(* Logix 5000 Program export KEP; software revision 30.00; part 7 of 15 *)

ADD_ON_INSTRUCTION B256_DEC   (* revision 1.0 20170916, vendor Kenneth A. Fischer *)
// c1 = --c1
// Revision note:
// Rev1.0: 20170916 - Initial Release
VAR_IN_OUT
   Inp_C : DINT[22]; {required}
END_VAR
VAR
   i : DINT;
END_VAR

ROUTINE Logic   (* ladder *)
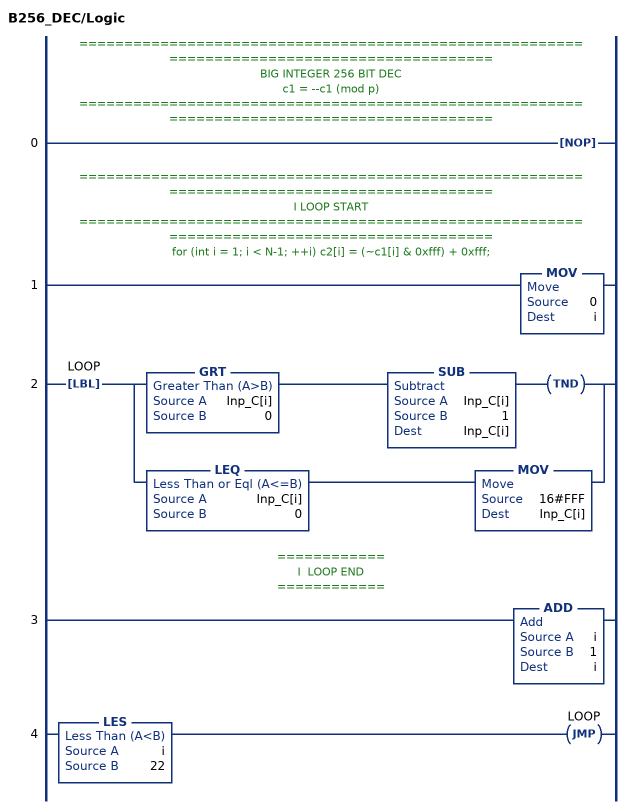
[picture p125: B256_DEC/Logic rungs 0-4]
   // ============================================================================================
   // BIG INTEGER 256 BIT DEC
   // c1 = --c1 (mod p)
   // ============================================================================================
   0: NOP();
   // ============================================================================================
   // I LOOP START
   // ============================================================================================
   // for (int i = 1; i < N-1; ++i) c2[i] = (~c1[i] & 0xfff) + 0xfff;
   1: MOV(0,i);
   2: LBL(LOOP)[GRT(Inp_C[i],0) SUB(Inp_C[i],1,Inp_C[i]) TND() ,LEQ(Inp_C[i],0) MOV(16#FFF,Inp_C[i]) ];
   // ============
   // I  LOOP END
   // ============
   3: ADD(i,1,i);
   4: LES(i,22)JMP(LOOP);
END_ROUTINE
END_ADD_ON_INSTRUCTION

ADD_ON_INSTRUCTION B256_MODPOW   (* revision 1.0 20170916, vendor Kenneth A. Fischer *)
// c2 = c1^e mod (2^255-19)
// Revision note:
// Rev1.0: 20170916 - Initial Release
VAR_IN_OUT
   Temp_C1 : DINT[22]; {required}
   Temp_C2 : DINT[22]; {required}
   Temp_D : DINT[43]; {required}
   Inp_C1 : DINT[22]; {required}   // V
   Inp_E : DINT[32]; {required}
   Out_C2 : DINT[22]; {required}   // U
END_VAR
VAR_OUTPUT
   i : INT; {access Read Only}
END_VAR
VAR_INPUT
   SEQCTRL_RESET : BOOL;   // Resets Point Multiplication if Toggled True
END_VAR
VAR_OUTPUT
   SEQCTRL_DN : BOOL; {access Read Only}   // Complete
   SEQCTRL_STEP : INT; {access Read Only}
END_VAR
VAR
   SEQCTRL_CMD : INT;
   SEQCTRL_DONE : INT;
   SEQCTRL_CMD_TABLE : INT[35];
   SEQCTRL_NEXT_STEP : INT;
   TEMP : INT;
   j : INT;
   b : DINT;
   B256_MUL : B256_MUL;
   B256_SQU : B256_SQU;
END_VAR

ROUTINE Logic   (* ladder *)
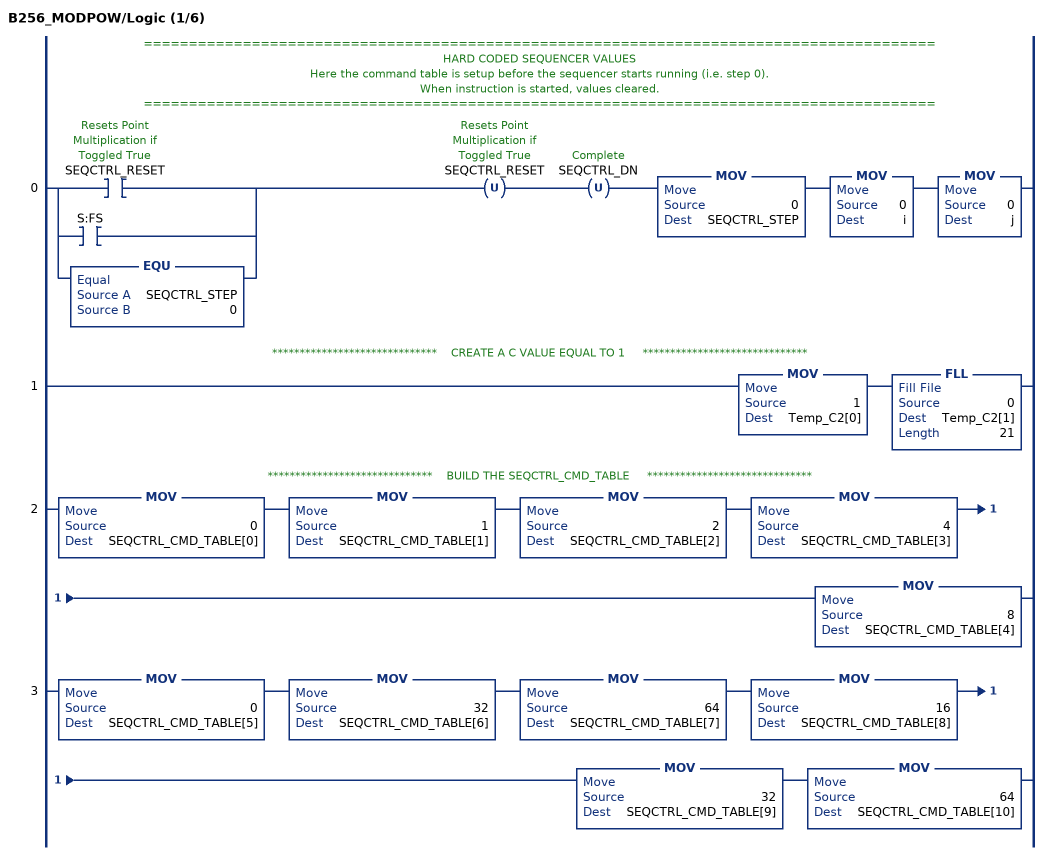
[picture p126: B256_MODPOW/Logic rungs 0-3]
   // ========================================================================================
   // HARD CODED SEQUENCER VALUES
   // Here the command table is setup before the sequencer starts running (i.e. step 0).
   // When instruction is started, values cleared.
   // ========================================================================================
   0: [[XIC(SEQCTRL_RESET) ,XIC(S:FS) ] ,EQU(SEQCTRL_STEP,0) ]OTU(SEQCTRL_RESET)OTU(SEQCTRL_DN)MOV(0,SEQCTRL_STEP)MOV(0,i)MOV(0,j);
   // ******************************    CREATE A C VALUE EQUAL TO 1     ******************************
   1: MOV(1,Temp_C2[0])FLL(0,Temp_C2[1],21);
   // ******************************    BUILD THE SEQCTRL_CMD_TABLE     ******************************
   2: MOV(0,SEQCTRL_CMD_TABLE[0])MOV(1,SEQCTRL_CMD_TABLE[1])MOV(2,SEQCTRL_CMD_TABLE[2])MOV(4,SEQCTRL_CMD_TABLE[3])MOV(8,SEQCTRL_CMD_TABLE[4]);
   3: MOV(0,SEQCTRL_CMD_TABLE[5])MOV(32,SEQCTRL_CMD_TABLE[6])MOV(64,SEQCTRL_CMD_TABLE[7])MOV(16,SEQCTRL_CMD_TABLE[8])MOV(32,SEQCTRL_CMD_TABLE[9])MOV(64,SEQCTRL_CMD_TABLE[10]);
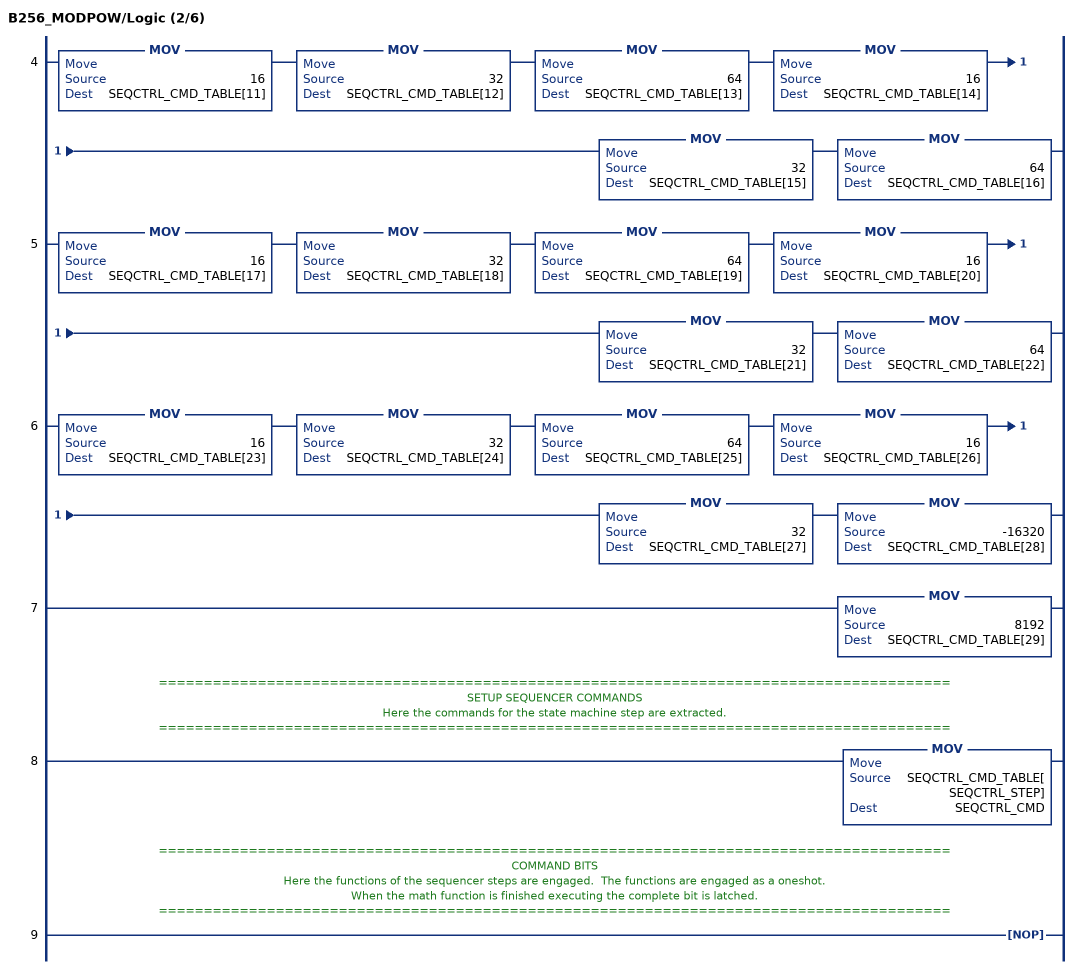
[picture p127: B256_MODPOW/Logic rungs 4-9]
   4: MOV(16,SEQCTRL_CMD_TABLE[11])MOV(32,SEQCTRL_CMD_TABLE[12])MOV(64,SEQCTRL_CMD_TABLE[13])MOV(16,SEQCTRL_CMD_TABLE[14])MOV(32,SEQCTRL_CMD_TABLE[15])MOV(64,SEQCTRL_CMD_TABLE[16]);
   5: MOV(16,SEQCTRL_CMD_TABLE[17])MOV(32,SEQCTRL_CMD_TABLE[18])MOV(64,SEQCTRL_CMD_TABLE[19])MOV(16,SEQCTRL_CMD_TABLE[20])MOV(32,SEQCTRL_CMD_TABLE[21])MOV(64,SEQCTRL_CMD_TABLE[22]);
   6: MOV(16,SEQCTRL_CMD_TABLE[23])MOV(32,SEQCTRL_CMD_TABLE[24])MOV(64,SEQCTRL_CMD_TABLE[25])MOV(16,SEQCTRL_CMD_TABLE[26])MOV(32,SEQCTRL_CMD_TABLE[27])MOV(-16320,SEQCTRL_CMD_TABLE[28]);
   7: MOV(8192,SEQCTRL_CMD_TABLE[29]);
   // ========================================================================================
   // SETUP SEQUENCER COMMANDS
   // Here the commands for the state machine step are extracted.
   // ========================================================================================
   8: MOV(SEQCTRL_CMD_TABLE[SEQCTRL_STEP],SEQCTRL_CMD);
   // ========================================================================================
   // COMMAND BITS
   // Here the functions of the sequencer steps are engaged.  The functions are engaged as a oneshot.
   // When the math function is finished executing the complete bit is latched.
   // ========================================================================================
   9: NOP();
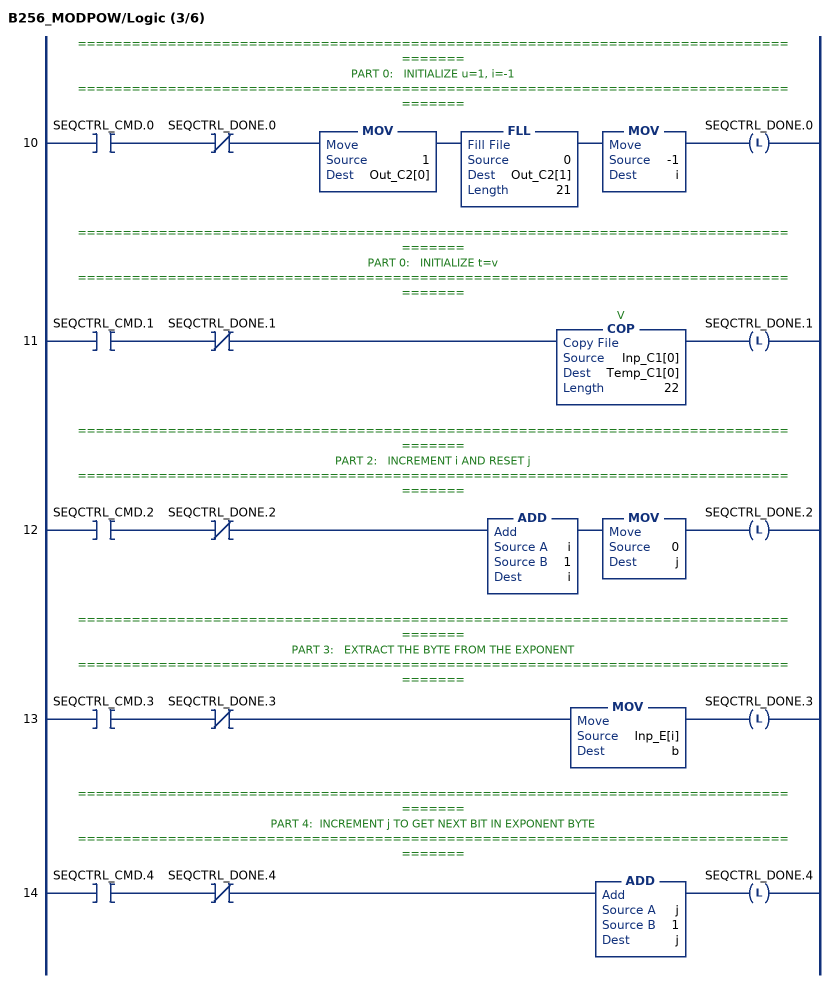
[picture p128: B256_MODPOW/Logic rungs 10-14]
   // ======================================================================================
   // PART 0:   INITIALIZE u=1, i=-1
   // ======================================================================================
   10: XIC(SEQCTRL_CMD.0)XIO(SEQCTRL_DONE.0)MOV(1,Out_C2[0])FLL(0,Out_C2[1],21)MOV(-1,i)OTL(SEQCTRL_DONE.0);
   // ======================================================================================
   // PART 0:   INITIALIZE t=v
   // ======================================================================================
   11: XIC(SEQCTRL_CMD.1)XIO(SEQCTRL_DONE.1)COP(Inp_C1[0],Temp_C1[0],22)OTL(SEQCTRL_DONE.1);
   // ======================================================================================
   // PART 2:   INCREMENT i AND RESET j
   // ======================================================================================
   12: XIC(SEQCTRL_CMD.2)XIO(SEQCTRL_DONE.2)ADD(i,1,i)MOV(0,j)OTL(SEQCTRL_DONE.2);
   // ======================================================================================
   // PART 3:   EXTRACT THE BYTE FROM THE EXPONENT
   // ======================================================================================
   13: XIC(SEQCTRL_CMD.3)XIO(SEQCTRL_DONE.3)MOV(Inp_E[i],b)OTL(SEQCTRL_DONE.3);
   // ======================================================================================
   // PART 4:  INCREMENT j TO GET NEXT BIT IN EXPONENT BYTE
   // ======================================================================================
   14: XIC(SEQCTRL_CMD.4)XIO(SEQCTRL_DONE.4)ADD(j,1,j)OTL(SEQCTRL_DONE.4);
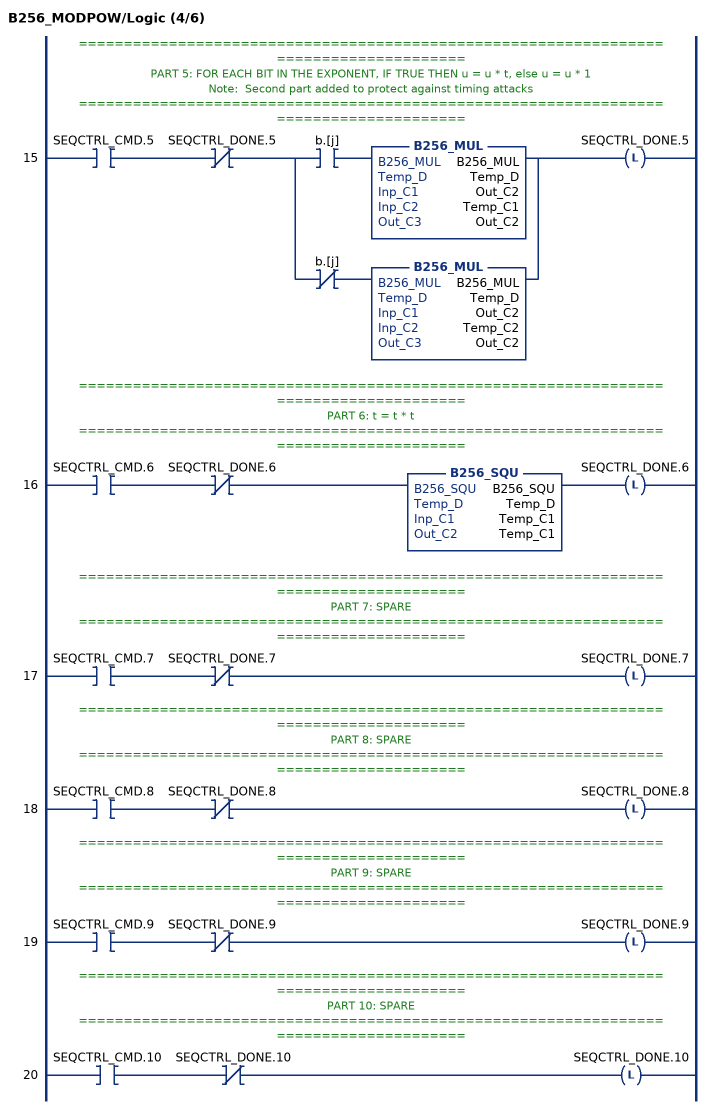
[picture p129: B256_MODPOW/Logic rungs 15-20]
   // ======================================================================================
   // PART 5: FOR EACH BIT IN THE EXPONENT, IF TRUE THEN u = u * t, else u = u * 1
   // Note:  Second part added to protect against timing attacks
   // ======================================================================================
   15: XIC(SEQCTRL_CMD.5)XIO(SEQCTRL_DONE.5)[XIC(b.[j]) B256_MUL(B256_MUL,Temp_D,Out_C2,Temp_C1,Out_C2) ,XIO(b.[j]) B256_MUL(B256_MUL,Temp_D,Out_C2,Temp_C2,Out_C2) ]OTL(SEQCTRL_DONE.5);
   // ======================================================================================
   // PART 6: t = t * t
   // ======================================================================================
   16: XIC(SEQCTRL_CMD.6)XIO(SEQCTRL_DONE.6)B256_SQU(B256_SQU,Temp_D,Temp_C1,Temp_C1)OTL(SEQCTRL_DONE.6);
   // ======================================================================================
   // PART 7: SPARE
   // ======================================================================================
   17: XIC(SEQCTRL_CMD.7)XIO(SEQCTRL_DONE.7)OTL(SEQCTRL_DONE.7);
   // ======================================================================================
   // PART 8: SPARE
   // ======================================================================================
   18: XIC(SEQCTRL_CMD.8)XIO(SEQCTRL_DONE.8)OTL(SEQCTRL_DONE.8);
   // ======================================================================================
   // PART 9: SPARE
   // ======================================================================================
   19: XIC(SEQCTRL_CMD.9)XIO(SEQCTRL_DONE.9)OTL(SEQCTRL_DONE.9);
   // ======================================================================================
   // PART 10: SPARE
   // ======================================================================================
   20: XIC(SEQCTRL_CMD.10)XIO(SEQCTRL_DONE.10)OTL(SEQCTRL_DONE.10);
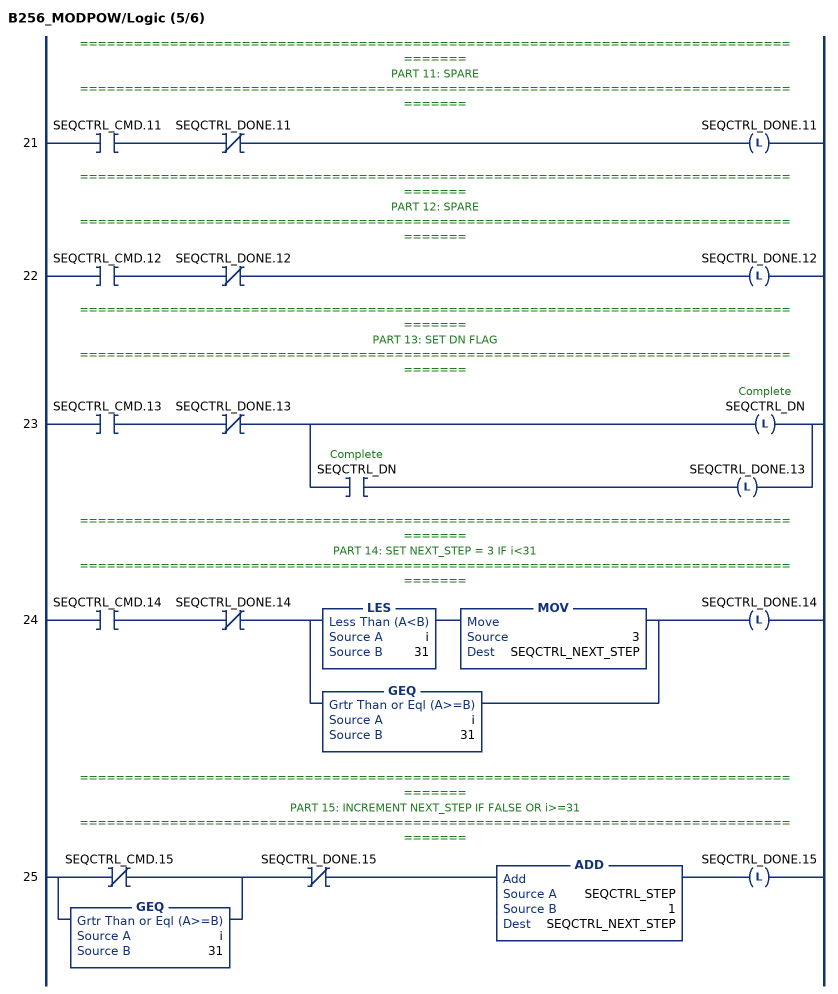
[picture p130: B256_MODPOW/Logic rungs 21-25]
   // ======================================================================================
   // PART 11: SPARE
   // ======================================================================================
   21: XIC(SEQCTRL_CMD.11)XIO(SEQCTRL_DONE.11)OTL(SEQCTRL_DONE.11);
   // ======================================================================================
   // PART 12: SPARE
   // ======================================================================================
   22: XIC(SEQCTRL_CMD.12)XIO(SEQCTRL_DONE.12)OTL(SEQCTRL_DONE.12);
   // ======================================================================================
   // PART 13: SET DN FLAG
   // ======================================================================================
   23: XIC(SEQCTRL_CMD.13)XIO(SEQCTRL_DONE.13)[OTL(SEQCTRL_DN) ,XIC(SEQCTRL_DN) OTL(SEQCTRL_DONE.13) ];
   // ======================================================================================
   // PART 14: SET NEXT_STEP = 3 IF i<31
   // ======================================================================================
   24: XIC(SEQCTRL_CMD.14)XIO(SEQCTRL_DONE.14)[LES(i,31) MOV(3,SEQCTRL_NEXT_STEP) ,GEQ(i,31) ]OTL(SEQCTRL_DONE.14);
   // ======================================================================================
   // PART 15: INCREMENT NEXT_STEP IF FALSE OR i>=31
   // ======================================================================================
   25: [XIO(SEQCTRL_CMD.15) ,GEQ(i,31) ]XIO(SEQCTRL_DONE.15)ADD(SEQCTRL_STEP,1,SEQCTRL_NEXT_STEP)OTL(SEQCTRL_DONE.15);
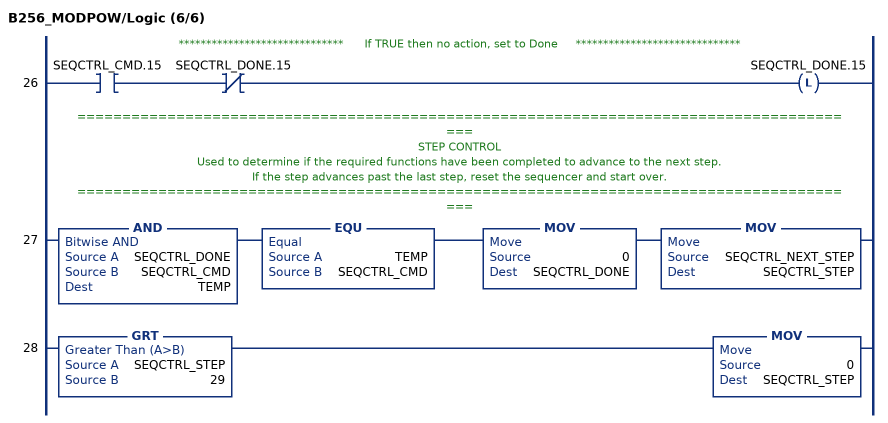
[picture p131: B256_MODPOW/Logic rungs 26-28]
   // ******************************      If TRUE then no action, set to Done     ******************************
   26: XIC(SEQCTRL_CMD.15)XIO(SEQCTRL_DONE.15)OTL(SEQCTRL_DONE.15);
   // ========================================================================================
   // STEP CONTROL
   // Used to determine if the required functions have been completed to advance to the next step.
   // If the step advances past the last step, reset the sequencer and start over.
   // ========================================================================================
   27: AND(SEQCTRL_DONE,SEQCTRL_CMD,TEMP)EQU(TEMP,SEQCTRL_CMD)MOV(0,SEQCTRL_DONE)MOV(SEQCTRL_NEXT_STEP,SEQCTRL_STEP);
   28: GRT(SEQCTRL_STEP,29)MOV(0,SEQCTRL_STEP);
END_ROUTINE
END_ADD_ON_INSTRUCTION

ADD_ON_INSTRUCTION B256_NEG   (* revision 1.0 20170916, vendor Kenneth A. Fischer *)
// c2 = -c1 (mod p)
// Revision note:
// Rev1.0: 20170916 - Initial Release
VAR_OUTPUT
   FAIL : BOOL; {access Read Only}   // Indicates negative overflow which should not happen
END_VAR
VAR_IN_OUT
   Inp_C1 : DINT[22]; {required}
   Out_C2 : DINT[22]; {required}
END_VAR
VAR
   s : DINT;
   b : DINT;
   i : DINT;
END_VAR

ROUTINE Logic   (* ladder *)
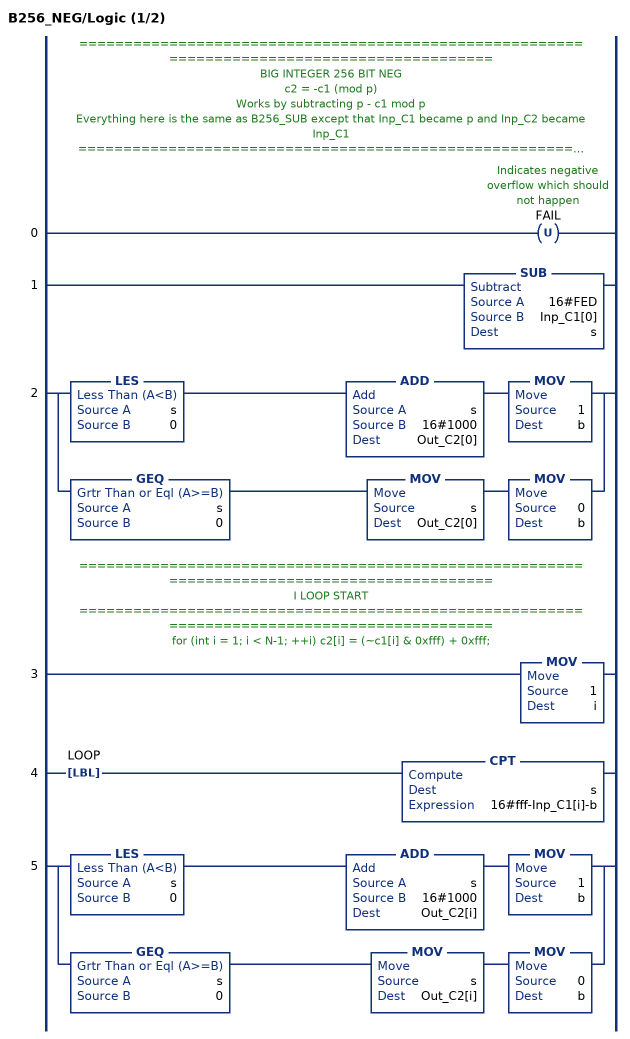
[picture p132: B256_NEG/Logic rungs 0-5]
   // ============================================================================================
   // BIG INTEGER 256 BIT NEG
   // c2 = -c1 (mod p)
   // Works by subtracting p - c1 mod p
   // Everything here is the same as B256_SUB except that Inp_C1 became p and Inp_C2 became Inp_C1
   // ============================================================================================
   0: OTU(FAIL);
   1: SUB(16#FED,Inp_C1[0],s);
   2: [LES(s,0) ADD(s,16#1000,Out_C2[0]) MOV(1,b) ,GEQ(s,0) MOV(s,Out_C2[0]) MOV(0,b) ];
   // ============================================================================================
   // I LOOP START
   // ============================================================================================
   // for (int i = 1; i < N-1; ++i) c2[i] = (~c1[i] & 0xfff) + 0xfff;
   3: MOV(1,i);
   4: LBL(LOOP)CPT(s,16#fff-Inp_C1[i]-b);
   5: [LES(s,0) ADD(s,16#1000,Out_C2[i]) MOV(1,b) ,GEQ(s,0) MOV(s,Out_C2[i]) MOV(0,b) ];
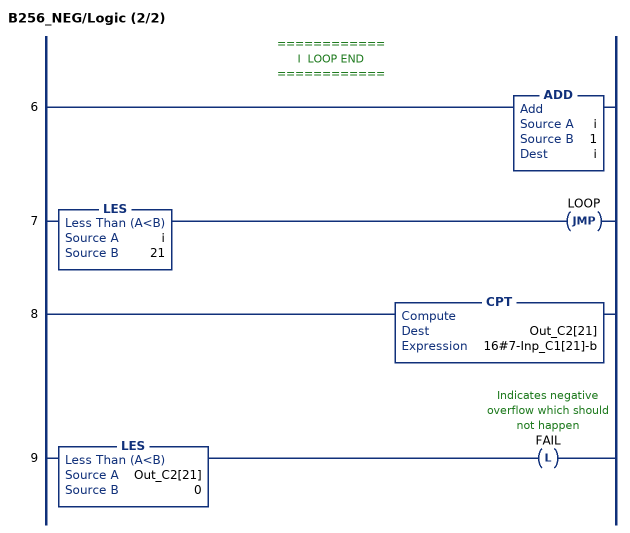
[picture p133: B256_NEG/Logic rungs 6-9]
   // ============
   // I  LOOP END
   // ============
   6: ADD(i,1,i);
   7: LES(i,21)JMP(LOOP);
   8: CPT(Out_C2[21],16#7-Inp_C1[21]-b);
   9: LES(Out_C2[21],0)OTL(FAIL);
END_ROUTINE
END_ADD_ON_INSTRUCTION

ADD_ON_INSTRUCTION POINT_DEC   (* revision 1.0 20170916, vendor Kenneth A. Fischer *)
// Point Decode:
// Decode a string value representing a point (x,y) into POINT data type in extended coordinates pieces
// Requires POINT UDT
// Revision note:
// Rev1.0: 20170916 - Initial Release
VAR_INPUT
   SEQCTRL_RESET : BOOL;   // Resets Point Multiplication if Toggled True
END_VAR
VAR_OUTPUT
   SEQCTRL_DN : BOOL; {access Read Only}   // Complete
   SEQCTRL_STEP : INT; {access Read Only}
   SEQCTRL_SUBSTEP : INT; {access Read Only}
   FAILED : BOOL; {access Read Only}
END_VAR
VAR_IN_OUT
   Temp_C1 : DINT[22]; {required}   // d
   Temp_C2 : DINT[22]; {required}   // m-1
   Temp_C3 : DINT[22]; {required}   // sqrtm1 = 2^((m-1)/4)
   Temp_C4 : DINT[22]; {required}   // u
   Temp_C5 : DINT[22]; {required}   // v
   Temp_C6 : DINT[22]; {required}   // v2
   Temp_C7 : DINT[22]; {required}   // v4
   Temp_C8 : DINT[22]; {required}   // t1
   Temp_C9 : DINT[22]; {required}   // t2
   Temp_C10 : DINT[22]; {required}   // t3
   Temp_C11 : DINT[22]; {required}
   Temp_C12 : DINT[22]; {required}
   Temp_D : DINT[43]; {required}
   Temp_E : DINT[32]; {required}   // m58 = (m-5)/8
   Inp_SLE : STRING; {required}   // Encoded Point as a String
   Out_P : POINT; {required}   // POINT in extended coordinates
END_VAR
VAR
   SEQCTRL_CMD : DINT;
   SEQCTRL_DONE : DINT;
   SEQCTRL_NEXT_STEP : INT;
   SEQCTRL_CMD_TABLE : DINT[40];
   TEMP : DINT;
   B256_StoC_LE : B256_StoC_LE;
   x_0 : BOOL;
   B256_SQU : B256_SQU;
   B256_SUB : B256_SUB;
   B256_MUL : B256_MUL;
   B256_ADD : B256_ADD;
   B256_MODPOW : B256_MODPOW;
   SEQCTRL_ONS : DINT;
   B256_COMPARE : B256_COMPARE;
   B256_NEG : B256_NEG;
   B256_COMPARE1 : B256_COMPARE;
   B256_COMPARE2 : B256_COMPARE;
   B256_ADJ : B256_ADJ;
   B256_DEC : B256_DEC;
END_VAR

ROUTINE Logic   (* ladder *)
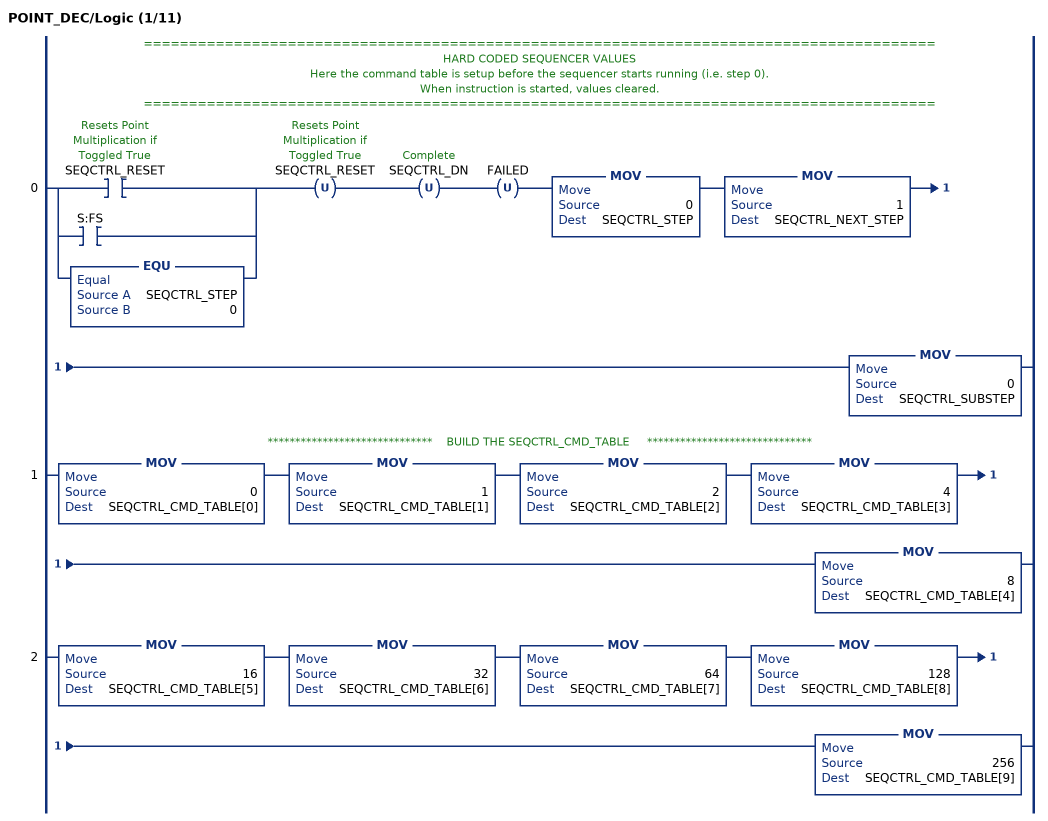
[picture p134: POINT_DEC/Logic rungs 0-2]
   // ========================================================================================
   // HARD CODED SEQUENCER VALUES
   // Here the command table is setup before the sequencer starts running (i.e. step 0).
   // When instruction is started, values cleared.
   // ========================================================================================
   0: [[XIC(SEQCTRL_RESET) ,XIC(S:FS) ] ,EQU(SEQCTRL_STEP,0) ]OTU(SEQCTRL_RESET)OTU(SEQCTRL_DN)OTU(FAILED)MOV(0,SEQCTRL_STEP)MOV(1,SEQCTRL_NEXT_STEP)MOV(0,SEQCTRL_SUBSTEP);
   // ******************************    BUILD THE SEQCTRL_CMD_TABLE     ******************************
   1: MOV(0,SEQCTRL_CMD_TABLE[0])MOV(1,SEQCTRL_CMD_TABLE[1])MOV(2,SEQCTRL_CMD_TABLE[2])MOV(4,SEQCTRL_CMD_TABLE[3])MOV(8,SEQCTRL_CMD_TABLE[4]);
   2: MOV(16,SEQCTRL_CMD_TABLE[5])MOV(32,SEQCTRL_CMD_TABLE[6])MOV(64,SEQCTRL_CMD_TABLE[7])MOV(128,SEQCTRL_CMD_TABLE[8])MOV(256,SEQCTRL_CMD_TABLE[9]);
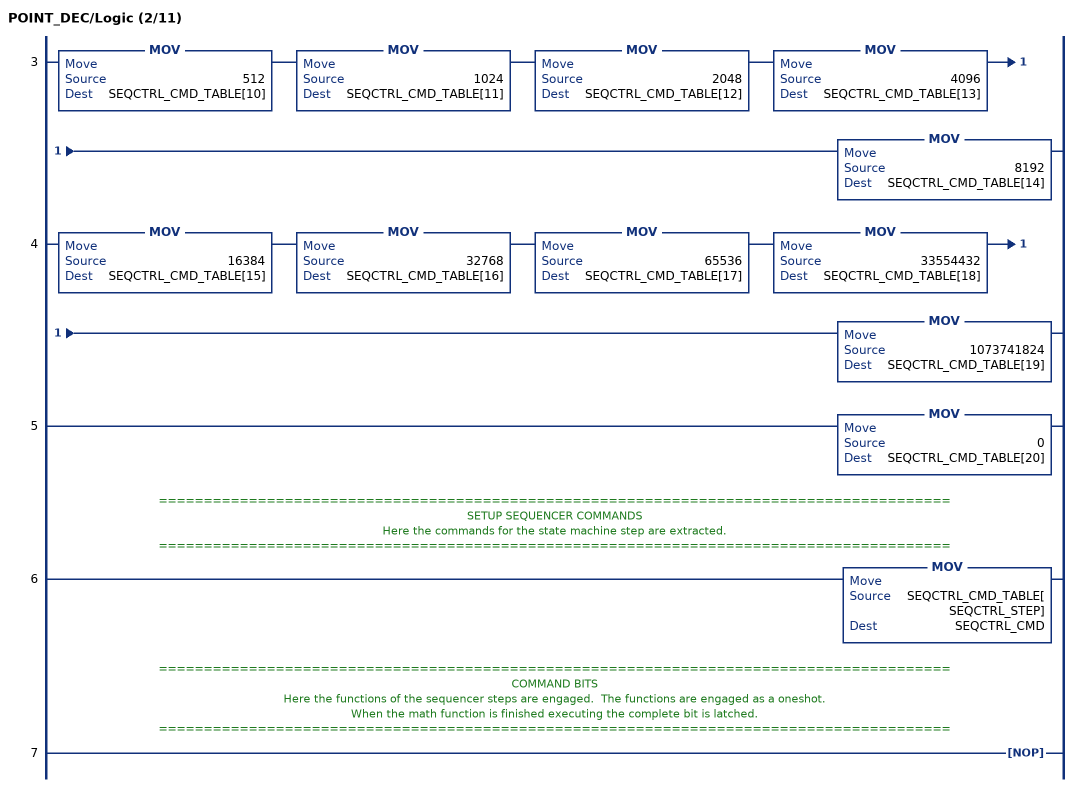
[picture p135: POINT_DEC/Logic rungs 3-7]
   3: MOV(512,SEQCTRL_CMD_TABLE[10])MOV(1024,SEQCTRL_CMD_TABLE[11])MOV(2048,SEQCTRL_CMD_TABLE[12])MOV(4096,SEQCTRL_CMD_TABLE[13])MOV(8192,SEQCTRL_CMD_TABLE[14]);
   4: MOV(16384,SEQCTRL_CMD_TABLE[15])MOV(32768,SEQCTRL_CMD_TABLE[16])MOV(65536,SEQCTRL_CMD_TABLE[17])MOV(33554432,SEQCTRL_CMD_TABLE[18])MOV(1073741824,SEQCTRL_CMD_TABLE[19]);
   5: MOV(0,SEQCTRL_CMD_TABLE[20]);
   // ========================================================================================
   // SETUP SEQUENCER COMMANDS
   // Here the commands for the state machine step are extracted.
   // ========================================================================================
   6: MOV(SEQCTRL_CMD_TABLE[SEQCTRL_STEP],SEQCTRL_CMD);
   // ========================================================================================
   // COMMAND BITS
   // Here the functions of the sequencer steps are engaged.  The functions are engaged as a oneshot.
   // When the math function is finished executing the complete bit is latched.
   // ========================================================================================
   7: NOP();
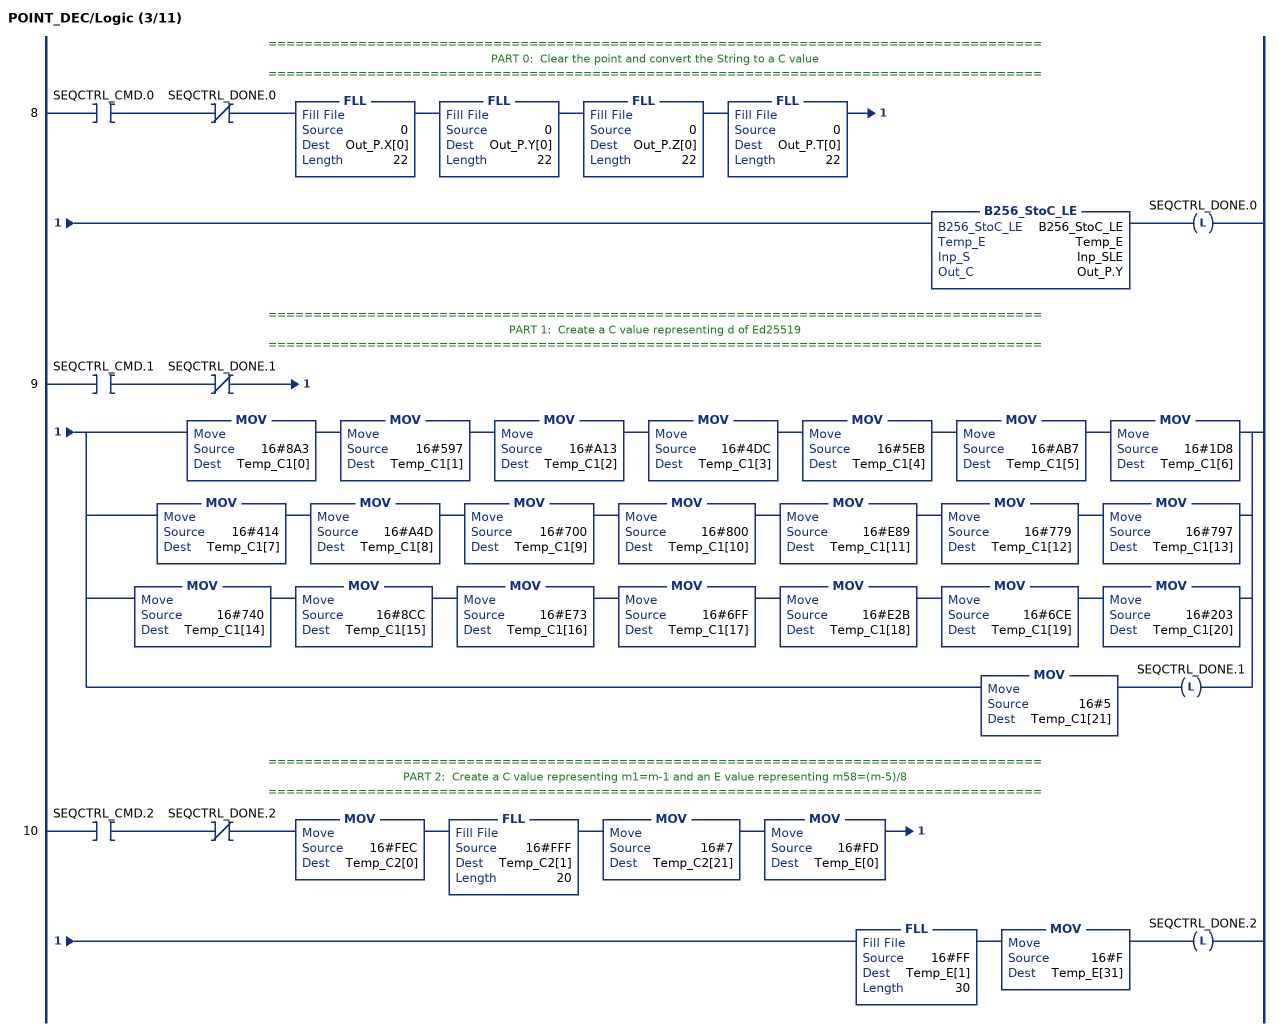
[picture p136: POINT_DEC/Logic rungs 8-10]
   // ======================================================================================
   // PART 0:  Clear the point and convert the String to a C value
   // ======================================================================================
   8: XIC(SEQCTRL_CMD.0)XIO(SEQCTRL_DONE.0)FLL(0,Out_P.X[0],22)FLL(0,Out_P.Y[0],22)FLL(0,Out_P.Z[0],22)FLL(0,Out_P.T[0],22)B256_StoC_LE(B256_StoC_LE,Temp_E,Inp_SLE,Out_P.Y)OTL(SEQCTRL_DONE.0);
   // ======================================================================================
   // PART 1:  Create a C value representing d of Ed25519
   // ======================================================================================
   9: XIC(SEQCTRL_CMD.1)XIO(SEQCTRL_DONE.1)[MOV(16#8A3,Temp_C1[0]) MOV(16#597,Temp_C1[1]) MOV(16#A13,Temp_C1[2]) MOV(16#4DC,Temp_C1[3]) MOV(16#5EB,Temp_C1[4]) MOV(16#AB7,Temp_C1[5]) MOV(16#1D8,Temp_C1[6]) ,MOV(16#414,Temp_C1[7]) MOV(16#A4D,Temp_C1[8]) MOV(16#700,Temp_C1[9]) MOV(16#800,Temp_C1[10]) MOV(16#E89,Temp_C1[11]) MOV(16#779,Temp_C1[12]) MOV(16#797,Temp_C1[13]) ,MOV(16#740,Temp_C1[14]) MOV(16#8CC,Temp_C1[15]) MOV(16#E73,Temp_C1[16]) MOV(16#6FF,Temp_C1[17]) MOV(16#E2B,Temp_C1[18]) MOV(16#6CE,Temp_C1[19]) MOV(16#203,Temp_C1[20]) ,MOV(16#5,Temp_C1[21]) OTL(SEQCTRL_DONE.1) ];
   // ======================================================================================
   // PART 2:  Create a C value representing m1=m-1 and an E value representing m58=(m-5)/8
   // ======================================================================================
   10: XIC(SEQCTRL_CMD.2)XIO(SEQCTRL_DONE.2)MOV(16#FEC,Temp_C2[0])FLL(16#FFF,Temp_C2[1],20)MOV(16#7,Temp_C2[21])MOV(16#FD,Temp_E[0])FLL(16#FF,Temp_E[1],30)MOV(16#F,Temp_E[31])OTL(SEQCTRL_DONE.2);
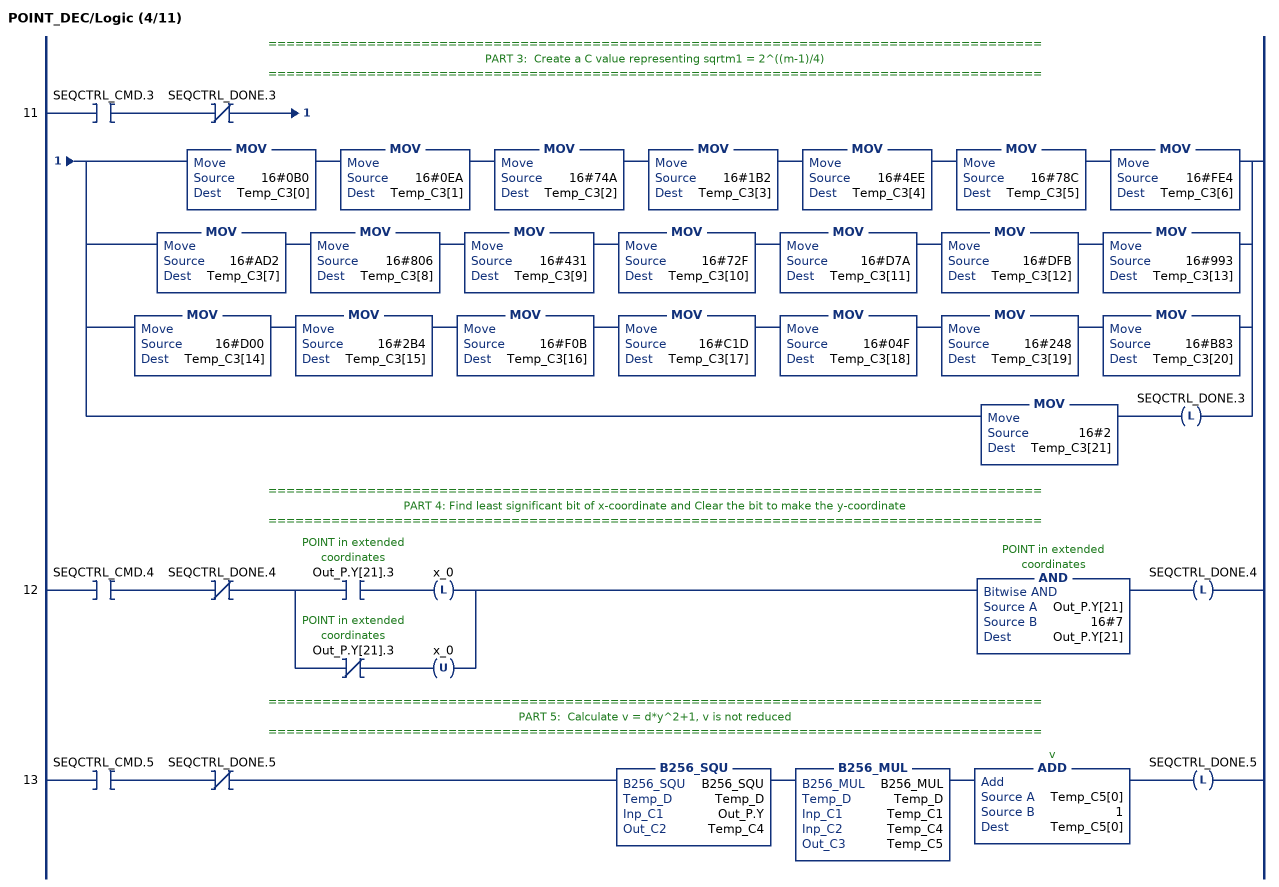
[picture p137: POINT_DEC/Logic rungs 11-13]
   // ======================================================================================
   // PART 3:  Create a C value representing sqrtm1 = 2^((m-1)/4)
   // ======================================================================================
   11: XIC(SEQCTRL_CMD.3)XIO(SEQCTRL_DONE.3)[MOV(16#0B0,Temp_C3[0]) MOV(16#0EA,Temp_C3[1]) MOV(16#74A,Temp_C3[2]) MOV(16#1B2,Temp_C3[3]) MOV(16#4EE,Temp_C3[4]) MOV(16#78C,Temp_C3[5]) MOV(16#FE4,Temp_C3[6]) ,MOV(16#AD2,Temp_C3[7]) MOV(16#806,Temp_C3[8]) MOV(16#431,Temp_C3[9]) MOV(16#72F,Temp_C3[10]) MOV(16#D7A,Temp_C3[11]) MOV(16#DFB,Temp_C3[12]) MOV(16#993,Temp_C3[13]) ,MOV(16#D00,Temp_C3[14]) MOV(16#2B4,Temp_C3[15]) MOV(16#F0B,Temp_C3[16]) MOV(16#C1D,Temp_C3[17]) MOV(16#04F,Temp_C3[18]) MOV(16#248,Temp_C3[19]) MOV(16#B83,Temp_C3[20]) ,MOV(16#2,Temp_C3[21]) OTL(SEQCTRL_DONE.3) ];
   // ======================================================================================
   // PART 4: Find least significant bit of x-coordinate and Clear the bit to make the y-coordinate
   // ======================================================================================
   12: XIC(SEQCTRL_CMD.4)XIO(SEQCTRL_DONE.4)[XIC(Out_P.Y[21].3) OTL(x_0) ,XIO(Out_P.Y[21].3) OTU(x_0) ]AND(Out_P.Y[21],16#7,Out_P.Y[21])OTL(SEQCTRL_DONE.4);
   // ======================================================================================
   // PART 5:  Calculate v = d*y^2+1, v is not reduced
   // ======================================================================================
   13: XIC(SEQCTRL_CMD.5)XIO(SEQCTRL_DONE.5)B256_SQU(B256_SQU,Temp_D,Out_P.Y,Temp_C4)B256_MUL(B256_MUL,Temp_D,Temp_C1,Temp_C4,Temp_C5)ADD(Temp_C5[0],1,Temp_C5[0])OTL(SEQCTRL_DONE.5);
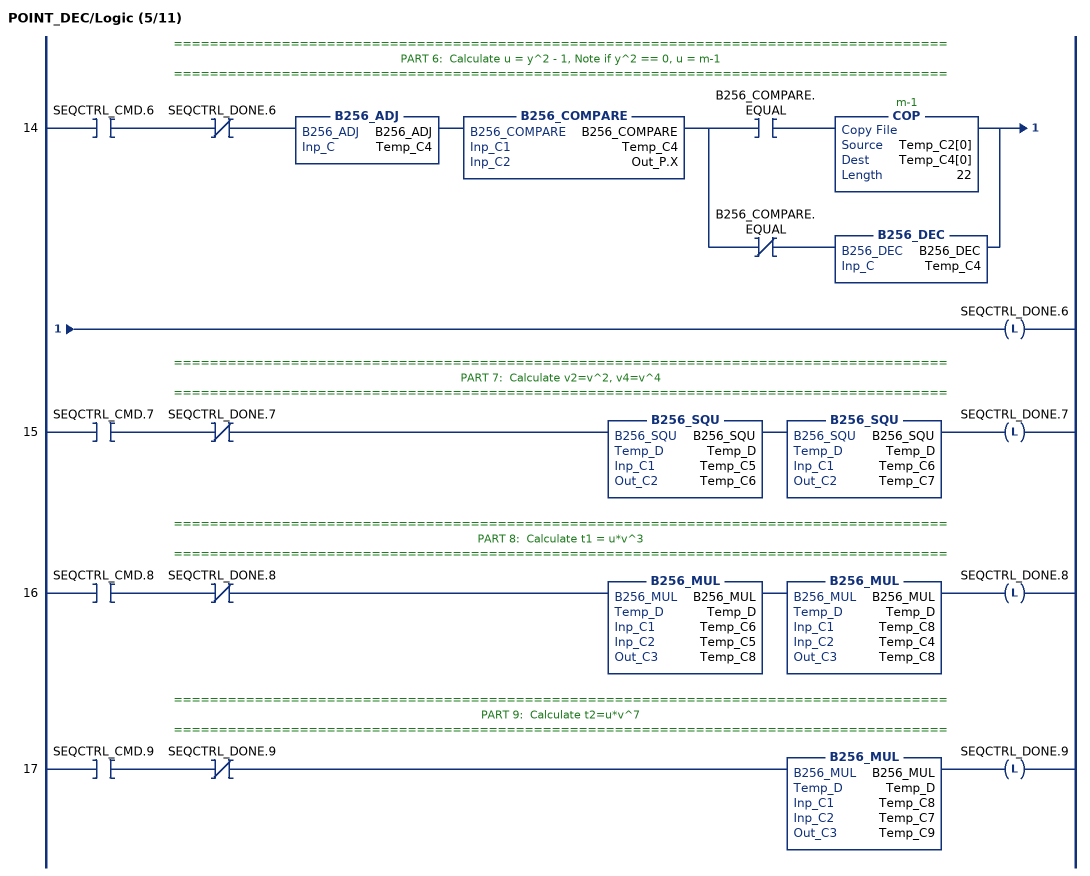
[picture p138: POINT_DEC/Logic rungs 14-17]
   // ======================================================================================
   // PART 6:  Calculate u = y^2 - 1, Note if y^2 == 0, u = m-1
   // ======================================================================================
   14: XIC(SEQCTRL_CMD.6)XIO(SEQCTRL_DONE.6)B256_ADJ(B256_ADJ,Temp_C4)B256_COMPARE(B256_COMPARE,Temp_C4,Out_P.X)[XIC(B256_COMPARE.EQUAL) COP(Temp_C2[0],Temp_C4[0],22) ,XIO(B256_COMPARE.EQUAL) B256_DEC(B256_DEC,Temp_C4) ]OTL(SEQCTRL_DONE.6);
   // ======================================================================================
   // PART 7:  Calculate v2=v^2, v4=v^4
   // ======================================================================================
   15: XIC(SEQCTRL_CMD.7)XIO(SEQCTRL_DONE.7)B256_SQU(B256_SQU,Temp_D,Temp_C5,Temp_C6)B256_SQU(B256_SQU,Temp_D,Temp_C6,Temp_C7)OTL(SEQCTRL_DONE.7);
   // ======================================================================================
   // PART 8:  Calculate t1 = u*v^3
   // ======================================================================================
   16: XIC(SEQCTRL_CMD.8)XIO(SEQCTRL_DONE.8)B256_MUL(B256_MUL,Temp_D,Temp_C6,Temp_C5,Temp_C8)B256_MUL(B256_MUL,Temp_D,Temp_C8,Temp_C4,Temp_C8)OTL(SEQCTRL_DONE.8);
   // ======================================================================================
   // PART 9:  Calculate t2=u*v^7
   // ======================================================================================
   17: XIC(SEQCTRL_CMD.9)XIO(SEQCTRL_DONE.9)B256_MUL(B256_MUL,Temp_D,Temp_C8,Temp_C7,Temp_C9)OTL(SEQCTRL_DONE.9);
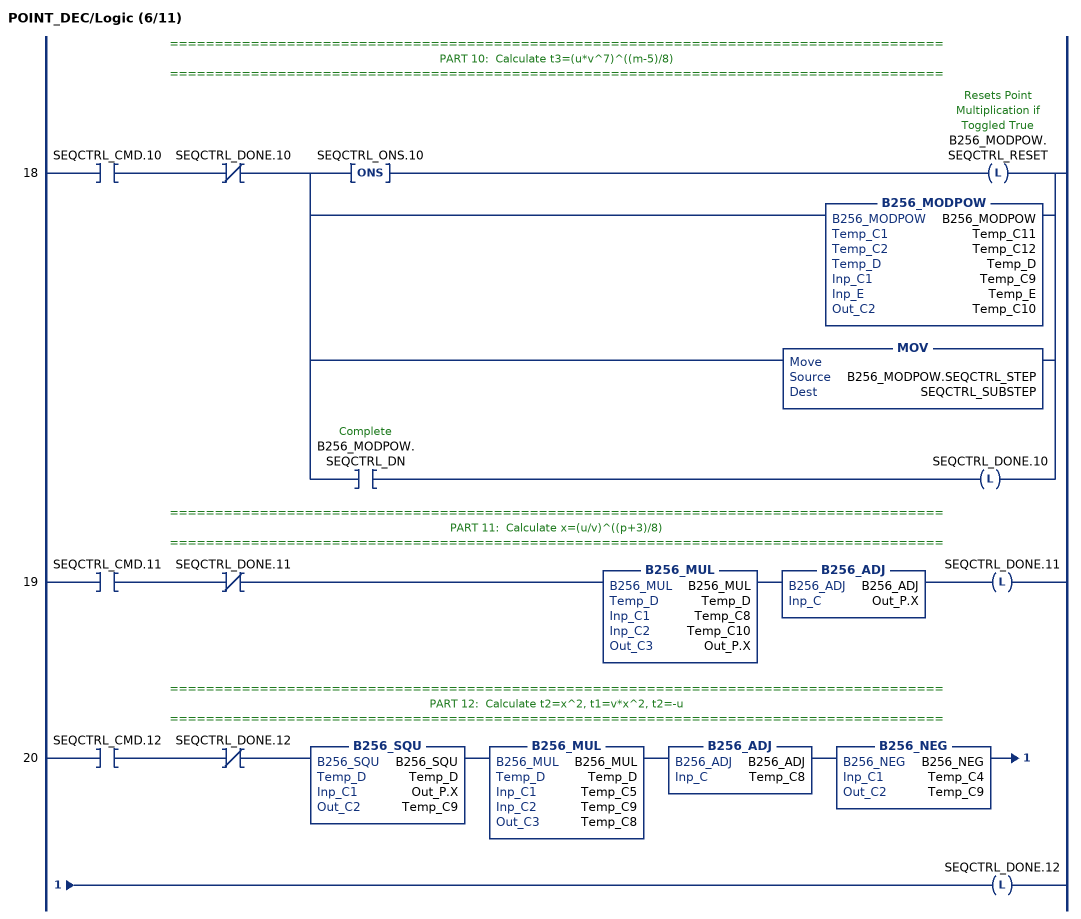
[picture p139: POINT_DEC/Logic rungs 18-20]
   // ======================================================================================
   // PART 10:  Calculate t3=(u*v^7)^((m-5)/8)
   // ======================================================================================
   18: XIC(SEQCTRL_CMD.10)XIO(SEQCTRL_DONE.10)[ONS(SEQCTRL_ONS.10) OTL(B256_MODPOW.SEQCTRL_RESET) ,B256_MODPOW(B256_MODPOW,Temp_C11,Temp_C12,Temp_D,Temp_C9,Temp_E,Temp_C10) ,MOV(B256_MODPOW.SEQCTRL_STEP,SEQCTRL_SUBSTEP) ,XIC(B256_MODPOW.SEQCTRL_DN) OTL(SEQCTRL_DONE.10) ];
   // ======================================================================================
   // PART 11:  Calculate x=(u/v)^((p+3)/8)
   // ======================================================================================
   19: XIC(SEQCTRL_CMD.11)XIO(SEQCTRL_DONE.11)B256_MUL(B256_MUL,Temp_D,Temp_C8,Temp_C10,Out_P.X)B256_ADJ(B256_ADJ,Out_P.X)OTL(SEQCTRL_DONE.11);
   // ======================================================================================
   // PART 12:  Calculate t2=x^2, t1=v*x^2, t2=-u
   // ======================================================================================
   20: XIC(SEQCTRL_CMD.12)XIO(SEQCTRL_DONE.12)B256_SQU(B256_SQU,Temp_D,Out_P.X,Temp_C9)B256_MUL(B256_MUL,Temp_D,Temp_C5,Temp_C9,Temp_C8)B256_ADJ(B256_ADJ,Temp_C8)B256_NEG(B256_NEG,Temp_C4,Temp_C9)OTL(SEQCTRL_DONE.12);
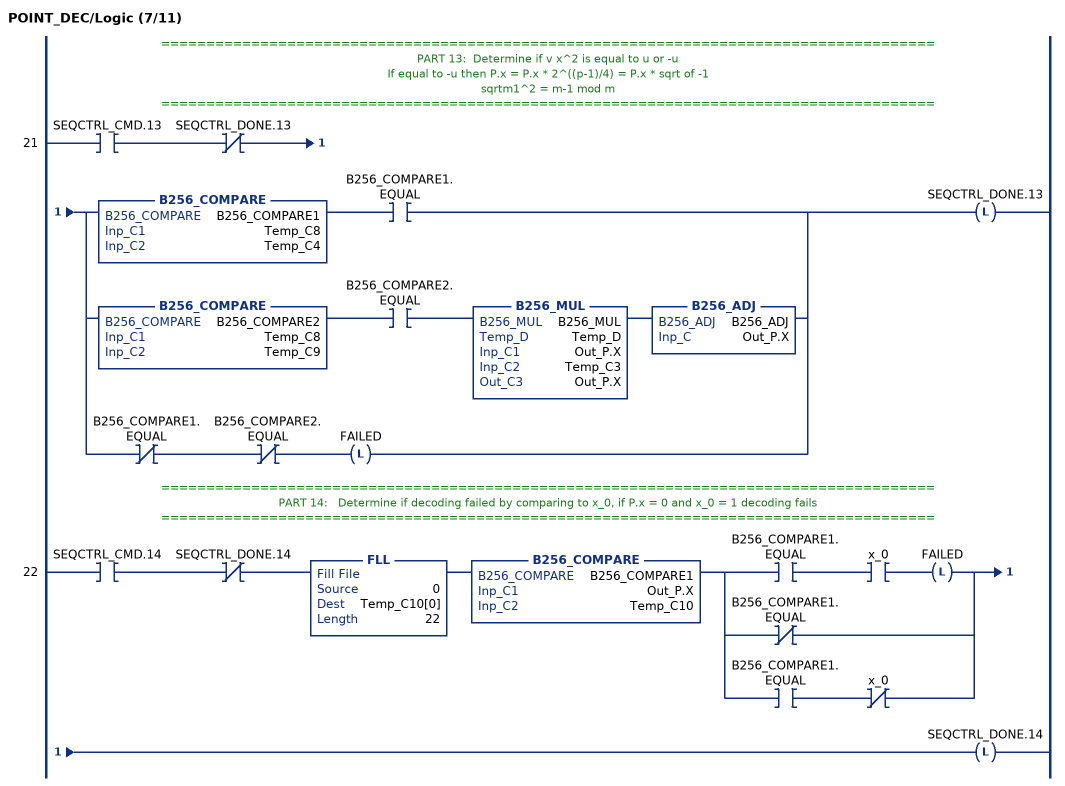
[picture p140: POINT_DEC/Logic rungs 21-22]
   // ======================================================================================
   // PART 13:  Determine if v x^2 is equal to u or -u
   // If equal to -u then P.x = P.x * 2^((p-1)/4) = P.x * sqrt of -1
   // sqrtm1^2 = m-1 mod m
   // ======================================================================================
   21: XIC(SEQCTRL_CMD.13)XIO(SEQCTRL_DONE.13)[B256_COMPARE(B256_COMPARE1,Temp_C8,Temp_C4) XIC(B256_COMPARE1.EQUAL) ,B256_COMPARE(B256_COMPARE2,Temp_C8,Temp_C9) XIC(B256_COMPARE2.EQUAL) B256_MUL(B256_MUL,Temp_D,Out_P.X,Temp_C3,Out_P.X) B256_ADJ(B256_ADJ,Out_P.X) ,XIO(B256_COMPARE1.EQUAL) XIO(B256_COMPARE2.EQUAL) OTL(FAILED) ]OTL(SEQCTRL_DONE.13);
   // ======================================================================================
   // PART 14:   Determine if decoding failed by comparing to x_0, if P.x = 0 and x_0 = 1 decoding fails
   // ======================================================================================
   22: XIC(SEQCTRL_CMD.14)XIO(SEQCTRL_DONE.14)FLL(0,Temp_C10[0],22)B256_COMPARE(B256_COMPARE1,Out_P.X,Temp_C10)[XIC(B256_COMPARE1.EQUAL) XIC(x_0) OTL(FAILED) ,XIO(B256_COMPARE1.EQUAL) ,XIC(B256_COMPARE1.EQUAL) XIO(x_0) ]OTL(SEQCTRL_DONE.14);
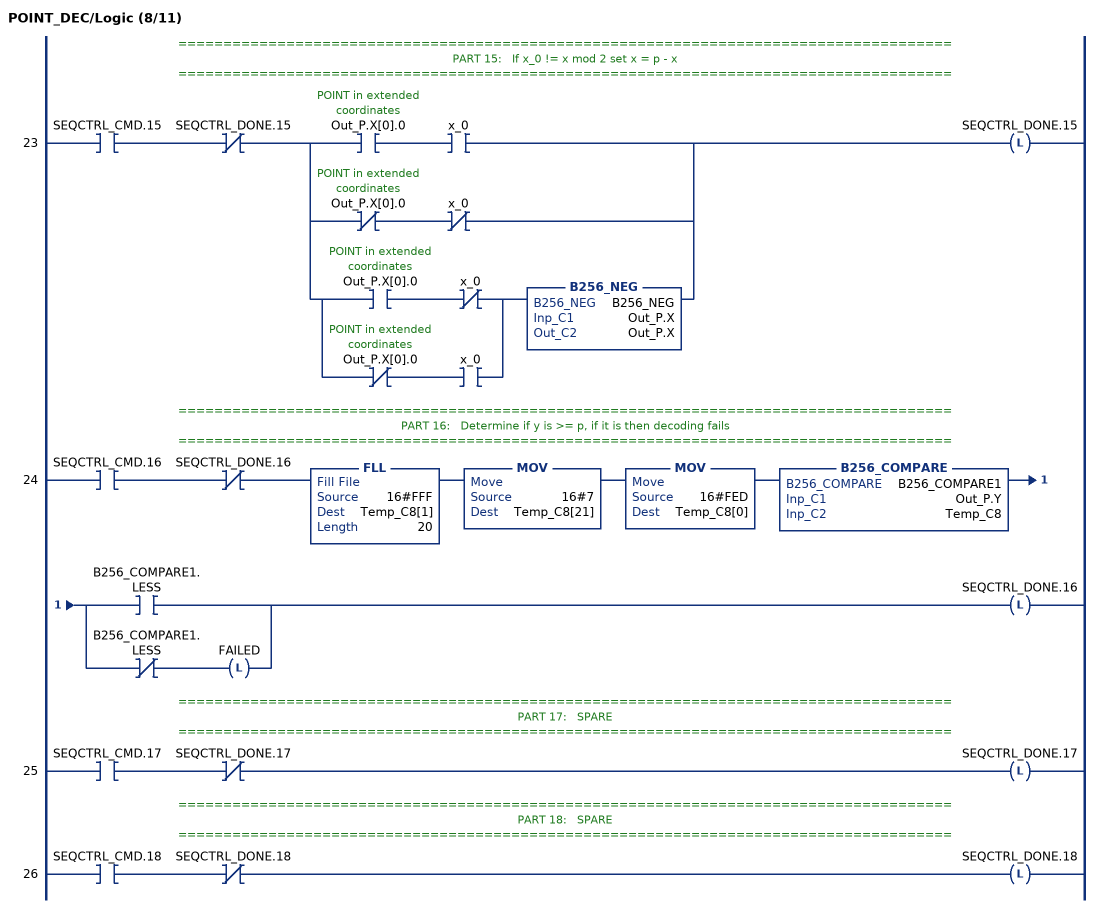
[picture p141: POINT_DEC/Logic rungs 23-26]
   // ======================================================================================
   // PART 15:   If x_0 != x mod 2 set x = p - x
   // ======================================================================================
   23: XIC(SEQCTRL_CMD.15)XIO(SEQCTRL_DONE.15)[XIC(Out_P.X[0].0) XIC(x_0) ,XIO(Out_P.X[0].0) XIO(x_0) ,[XIC(Out_P.X[0].0) XIO(x_0) ,XIO(Out_P.X[0].0) XIC(x_0) ] B256_NEG(B256_NEG,Out_P.X,Out_P.X) ]OTL(SEQCTRL_DONE.15);
   // ======================================================================================
   // PART 16:   Determine if y is >= p, if it is then decoding fails
   // ======================================================================================
   24: XIC(SEQCTRL_CMD.16)XIO(SEQCTRL_DONE.16)FLL(16#FFF,Temp_C8[1],20)MOV(16#7,Temp_C8[21])MOV(16#FED,Temp_C8[0])B256_COMPARE(B256_COMPARE1,Out_P.Y,Temp_C8)[XIC(B256_COMPARE1.LESS) ,XIO(B256_COMPARE1.LESS) OTL(FAILED) ]OTL(SEQCTRL_DONE.16);
   // ======================================================================================
   // PART 17:   SPARE
   // ======================================================================================
   25: XIC(SEQCTRL_CMD.17)XIO(SEQCTRL_DONE.17)OTL(SEQCTRL_DONE.17);
   // ======================================================================================
   // PART 18:   SPARE
   // ======================================================================================
   26: XIC(SEQCTRL_CMD.18)XIO(SEQCTRL_DONE.18)OTL(SEQCTRL_DONE.18);
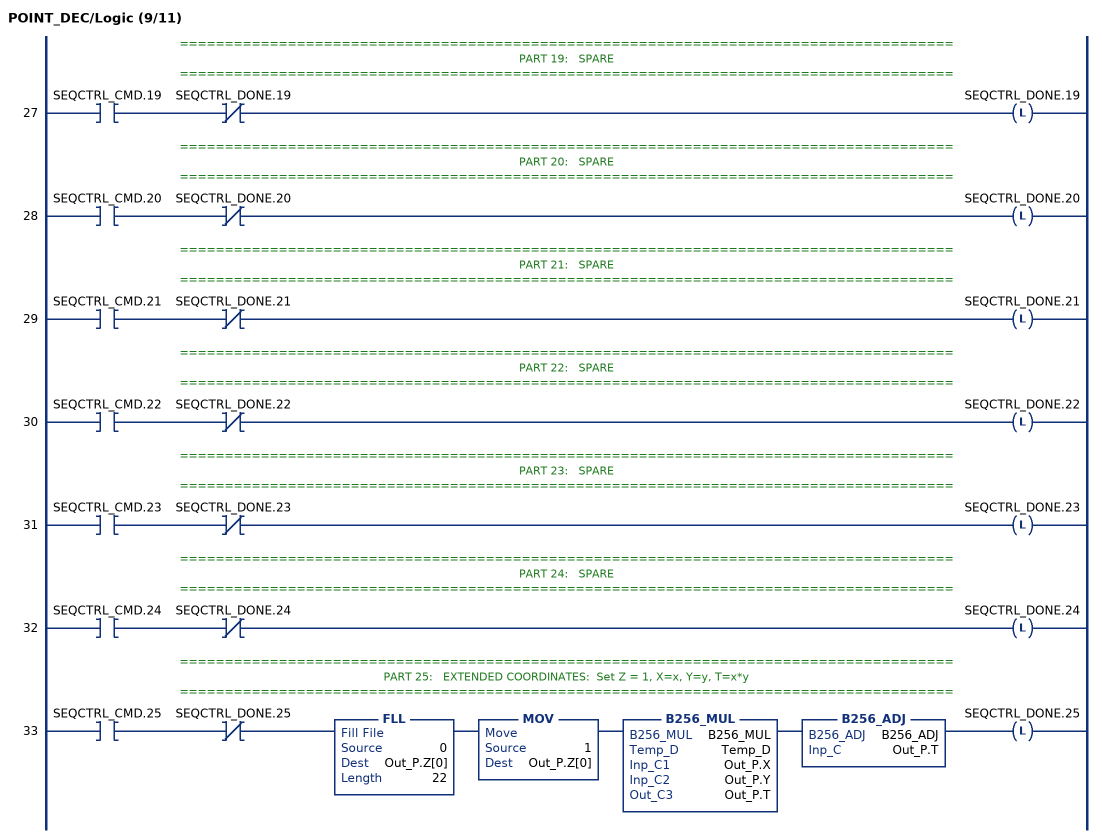
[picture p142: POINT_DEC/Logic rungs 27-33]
   // ======================================================================================
   // PART 19:   SPARE
   // ======================================================================================
   27: XIC(SEQCTRL_CMD.19)XIO(SEQCTRL_DONE.19)OTL(SEQCTRL_DONE.19);
   // ======================================================================================
   // PART 20:   SPARE
   // ======================================================================================
   28: XIC(SEQCTRL_CMD.20)XIO(SEQCTRL_DONE.20)OTL(SEQCTRL_DONE.20);
   // ======================================================================================
   // PART 21:   SPARE
   // ======================================================================================
   29: XIC(SEQCTRL_CMD.21)XIO(SEQCTRL_DONE.21)OTL(SEQCTRL_DONE.21);
   // ======================================================================================
   // PART 22:   SPARE
   // ======================================================================================
   30: XIC(SEQCTRL_CMD.22)XIO(SEQCTRL_DONE.22)OTL(SEQCTRL_DONE.22);
   // ======================================================================================
   // PART 23:   SPARE
   // ======================================================================================
   31: XIC(SEQCTRL_CMD.23)XIO(SEQCTRL_DONE.23)OTL(SEQCTRL_DONE.23);
   // ======================================================================================
   // PART 24:   SPARE
   // ======================================================================================
   32: XIC(SEQCTRL_CMD.24)XIO(SEQCTRL_DONE.24)OTL(SEQCTRL_DONE.24);
   // ======================================================================================
   // PART 25:   EXTENDED COORDINATES:  Set Z = 1, X=x, Y=y, T=x*y
   // ======================================================================================
   33: XIC(SEQCTRL_CMD.25)XIO(SEQCTRL_DONE.25)FLL(0,Out_P.Z[0],22)MOV(1,Out_P.Z[0])B256_MUL(B256_MUL,Temp_D,Out_P.X,Out_P.Y,Out_P.T)B256_ADJ(B256_ADJ,Out_P.T)OTL(SEQCTRL_DONE.25);
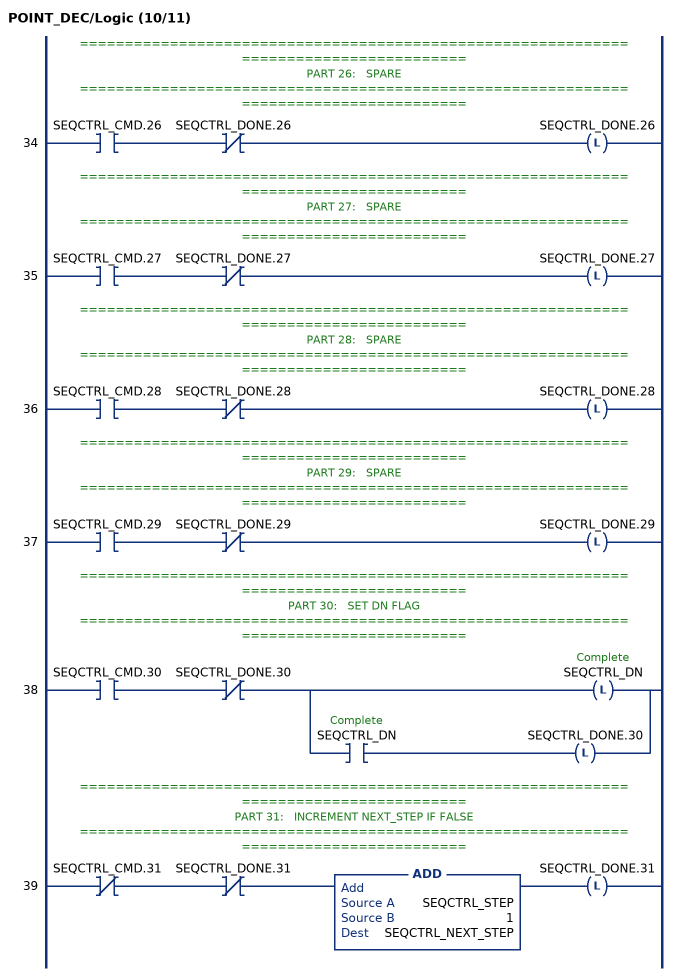
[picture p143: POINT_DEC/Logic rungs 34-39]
   // ======================================================================================
   // PART 26:   SPARE
   // ======================================================================================
   34: XIC(SEQCTRL_CMD.26)XIO(SEQCTRL_DONE.26)OTL(SEQCTRL_DONE.26);
   // ======================================================================================
   // PART 27:   SPARE
   // ======================================================================================
   35: XIC(SEQCTRL_CMD.27)XIO(SEQCTRL_DONE.27)OTL(SEQCTRL_DONE.27);
   // ======================================================================================
   // PART 28:   SPARE
   // ======================================================================================
   36: XIC(SEQCTRL_CMD.28)XIO(SEQCTRL_DONE.28)OTL(SEQCTRL_DONE.28);
   // ======================================================================================
   // PART 29:   SPARE
   // ======================================================================================
   37: XIC(SEQCTRL_CMD.29)XIO(SEQCTRL_DONE.29)OTL(SEQCTRL_DONE.29);
   // ======================================================================================
   // PART 30:   SET DN FLAG
   // ======================================================================================
   38: XIC(SEQCTRL_CMD.30)XIO(SEQCTRL_DONE.30)[OTL(SEQCTRL_DN) ,XIC(SEQCTRL_DN) OTL(SEQCTRL_DONE.30) ];
   // ======================================================================================
   // PART 31:   INCREMENT NEXT_STEP IF FALSE
   // ======================================================================================
   39: XIO(SEQCTRL_CMD.31)XIO(SEQCTRL_DONE.31)ADD(SEQCTRL_STEP,1,SEQCTRL_NEXT_STEP)OTL(SEQCTRL_DONE.31);
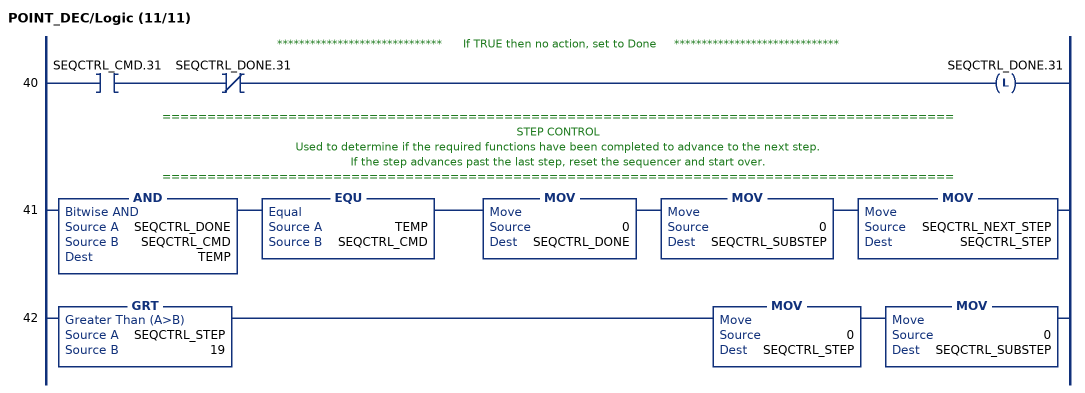
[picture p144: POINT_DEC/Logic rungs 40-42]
   // ******************************      If TRUE then no action, set to Done     ******************************
   40: XIC(SEQCTRL_CMD.31)XIO(SEQCTRL_DONE.31)OTL(SEQCTRL_DONE.31);
   // ========================================================================================
   // STEP CONTROL
   // Used to determine if the required functions have been completed to advance to the next step.
   // If the step advances past the last step, reset the sequencer and start over.
   // ========================================================================================
   41: AND(SEQCTRL_DONE,SEQCTRL_CMD,TEMP)EQU(TEMP,SEQCTRL_CMD)MOV(0,SEQCTRL_DONE)MOV(0,SEQCTRL_SUBSTEP)MOV(SEQCTRL_NEXT_STEP,SEQCTRL_STEP);
   42: GRT(SEQCTRL_STEP,19)MOV(0,SEQCTRL_STEP)MOV(0,SEQCTRL_SUBSTEP);
END_ROUTINE
END_ADD_ON_INSTRUCTION
